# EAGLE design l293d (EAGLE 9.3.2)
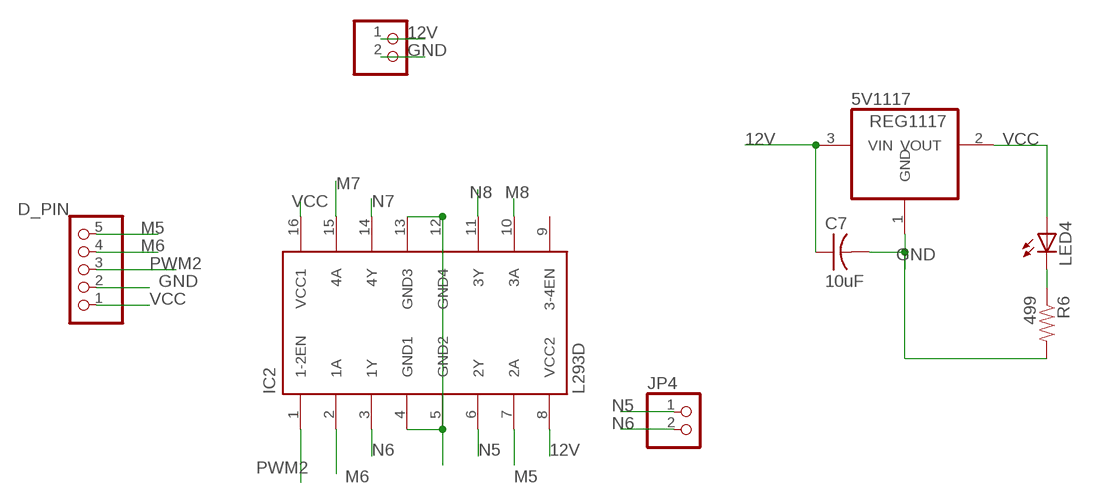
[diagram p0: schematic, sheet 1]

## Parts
5V1117  REG1117  [SOT223]
C7  10uF  CAP-US1206FAB  [C1206FAB]
D_PIN  PINHD-1X5  [1X05]
IC2  L293D  [DIL16]
JP3  PINHD-1X2  [1X02]
JP4  PINHD-1X2  [1X02]
LED4  LEDSMT1206  [1206]
R6  499  RESISTOR1206  [1206]

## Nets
12V: 5V1117.3(VIN) C7.1 IC2.8(VCC2) JP3.1
GND: 5V1117.1(GND) C7.2 D_PIN.2 IC2.4(GND1) IC2.5(GND2) IC2.12(GND4) IC2.13(GND3) JP3.2 R6.2
M5: D_PIN.5 IC2.7(2A)
M6: D_PIN.4 IC2.2(1A)
M7: IC2.15(4A)
M8: IC2.10(3A)
N5: IC2.6(2Y) JP4.1
N6: IC2.3(1Y) JP4.2
N7: IC2.14(4Y)
N8: IC2.11(3Y)
N$4: LED4.C R6.1
PWM2: D_PIN.3 IC2.1(1-2EN)
VCC: 5V1117.2(VOUT) D_PIN.1 IC2.16(VCC1) LED4.A
Unconnected: IC2.9(3-4EN)

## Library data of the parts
5V1117 = burr-brown:REG1117: 800mA and 1A Low Dropout (LDO) Positive Regulator 1.8V, 2.5V, 2.85V, 3.3V, 5V, and Adj; MPN: REG1117; OC_FARNELL: 1097566; OC_NEWARK: 14P6981
C7 = fab (1):CAP-US
D_PIN = pinhead:PINHD-1X5: PIN HEADER
IC2 = st-microelectronics:L293D: PUSH-PULL 4 CHANNEL DRIVER; MPN: L293D; OC_FARNELL: 9589619; OC_NEWARK: 56P8249
JP3 JP4 = pinhead:PINHD-1X2: PIN HEADER
LED4 = led:LED: LED
R6 = 01_SparkFun:RESISTOR: Resistor

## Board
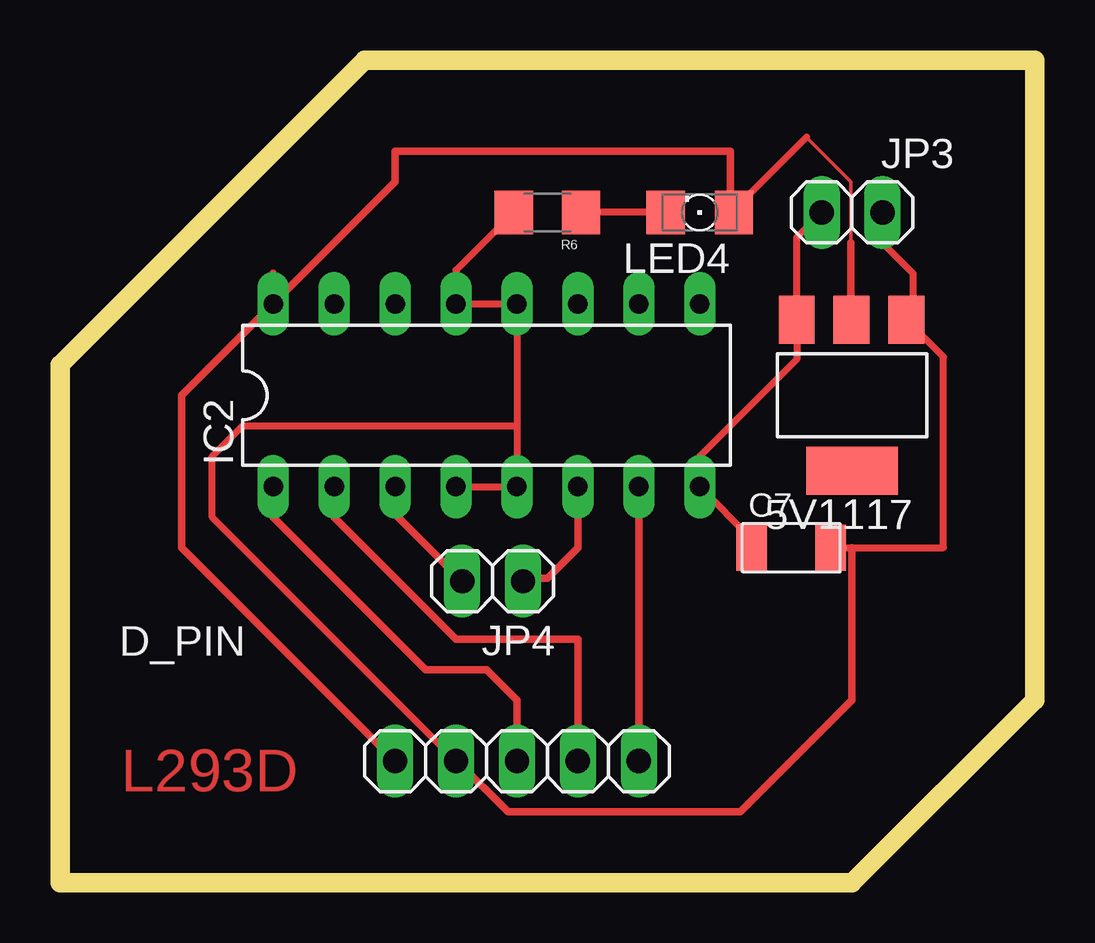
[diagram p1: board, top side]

Size 40.64 x 34.29 mm. Coordinates in mm from the lower left corner, seen from the top.
Outline: 12.7,34.29 0,21.59 0,0 33.02,0 40.64,7.62 40.64,34.29 12.7,34.29
Copper layers (1*16): Top 0.035mm / dielectric 1.5mm / Bottom 0.035mm
Design rules "fab (1) *": minimum track width 0.3mm, minimum drill 32mil, track to track 0.315mm, track to pad 0.315mm, pad to pad 0.315mm, via to via 0.315mm, smd to smd 0.315mm, copper to edge 40mil, drill to drill 16mil, minimum pad ring 10mil, minimum via ring 8mil, stop-mask expansion 4mil, vias tented up to drill 0mil, thermal gap 10mil

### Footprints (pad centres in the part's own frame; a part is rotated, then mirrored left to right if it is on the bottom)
SOT223 = smd 1.499 x 2.007: 1 -2.261,-3.15; 2 0.025,-3.15; 3 2.311,-3.15 | smd 3.81 x 2.007: 4 0,3.15
C1206FAB = smd 1.27 x 1.905: 1 -1.651,0; 2 1.651,0
1X05 = drill 1.016 long: 1 -5.08,0; 2 -2.54,0; 3 0,0; 4 2.54,0; 5 5.08,0
DIL16 = drill 0.813 long: 1 -8.89,-3.81; 2 -6.35,-3.81; 3 -3.81,-3.81; 4 -1.27,-3.81; 5 1.27,-3.81; 6 3.81,-3.81; 7 6.35,-3.81; 8 8.89,-3.81; 9 8.89,3.81; 10 6.35,3.81; 11 3.81,3.81; 12 1.27,3.81; 13 -1.27,3.81; 14 -3.81,3.81; 15 -6.35,3.81; 16 -8.89,3.81
1X02 = drill 1.016 long: 1 -1.27,0; 2 1.27,0
1206 = smd 1.6 x 1.803: A -1.422,0; C 1.422,0
1206' = smd 1.6 x 1.8: 1 -1.4,0; 2 1.4,0

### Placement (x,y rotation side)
5V1117  33.02,20.32 180 top
C7  30.48,13.97 0 top
D_PIN  19.05,5.08 0 top
IC2  17.78,20.32 0 top
JP3  33.02,27.94 0 top
JP4  18.03,12.57 180 top
LED4  26.67,27.94 180 top
R6  499  [1206']  20.32,27.94 180 top

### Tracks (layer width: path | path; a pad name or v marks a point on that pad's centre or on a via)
12V
  Top 0.3: C7.1 28.83,14.35 IC2.8 26.67,17.78 30.71,21.82 5V1117.3 30.71,26.9 JP3.1
GND
  Top 0.3: R6.2 16.51,25.53 IC2.13 IC2.12 19.05,19.05 | 19.05,19.05 IC2.5 IC2.4 | C7.2 33.02,13.97 36.83,13.97 36.83,21.92 35.56,23.19 | 35.56,23.19 5V1117.1 | JP3.2 34.29,26.67 35.56,25.4 35.56,23.19 | D_PIN.2 6.35,15.24 6.35,17.78 7.62,19.05 19.05,19.05
  Top 0.305: D_PIN.2 16.55,5.08 18.67,2.96 28.36,2.96 33.02,7.62 33.02,13.97
M5
  Top 0.305: IC2.7 D_PIN.5
M6
  Top 0.305: D_PIN.4 21.59,10.16 16.51,10.16 11.43,15.24 IC2.2
N5
  Top 0.305: IC2.6 21.59,13.97 20.32,12.7 19.43,12.7 JP4.1
N6
  Top 0.305: IC2.3 13.97,15.37 JP4.2
N$4
  Top 0.3: R6.1 LED4.C 25.4,27.94
PWM2
  Top 0.305: D_PIN.3 19.05,7.62 17.78,8.89 15.24,8.89 8.89,15.24 IC2.1
VCC
  Top 0.15: 31.12,31.07 32.98,29.21 32.98,26.67
  Top 0.3: 31.12,31.07 28.09,28.05 LED4.A | 5V1117.2 32.98,23.49
  Top 0.305: 32.98,23.49 32.98,26.67 | 8.89,25.4 IC2.16 | IC2.16 13.97,29.21 13.97,30.48 27.94,30.48 27.94,28.09 LED4.A | IC2.16 5.08,20.32 5.08,13.97 D_PIN.1

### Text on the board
Top: L293D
